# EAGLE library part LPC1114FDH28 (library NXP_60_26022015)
32-bit ARM Cortex-M0 microcontroller; up to 64 kB flash and 8 kB SRAM The LPC1110/11/12/13/14/15 are a ARM Cortex-M0 based, low-cost 32-bit MCU family, designed for 8/16-bit microcontroller applications, offering performance, low power, simple instruction set and memory addressing together with reduced code size compared to existing 8/16-bit architectures. The LPC1110/11/12/13/14/15 operate at CPU frequencies of up to 50 MHz. The peripheral complement of the LPC1110/11/12/13/14/15 includes up to 64 kB of flash memory, up to 8 kB of data memory, one Fast-mode Plus I 2 C-bus interface, one RS-485/EIA-485 UART, up to two SPI interfaces with SSP features, four general purpose counter/timers, a 10-bit ADC, and up to 42 general purpose I/O pins. Remark: The LPC111x series consists of the LPC1100 series (parts LPC111x/101/201/301), LPC1100L series (parts LPC111x/002/102/202/302), and the LPC1100XL series (parts LPC111x/103/203/303/323/333). The LPC1100L and LPC1100XL series include the power profiles, a windowed watchdog timer, and a configurable open-drain mode. AAL Eindhoven MK
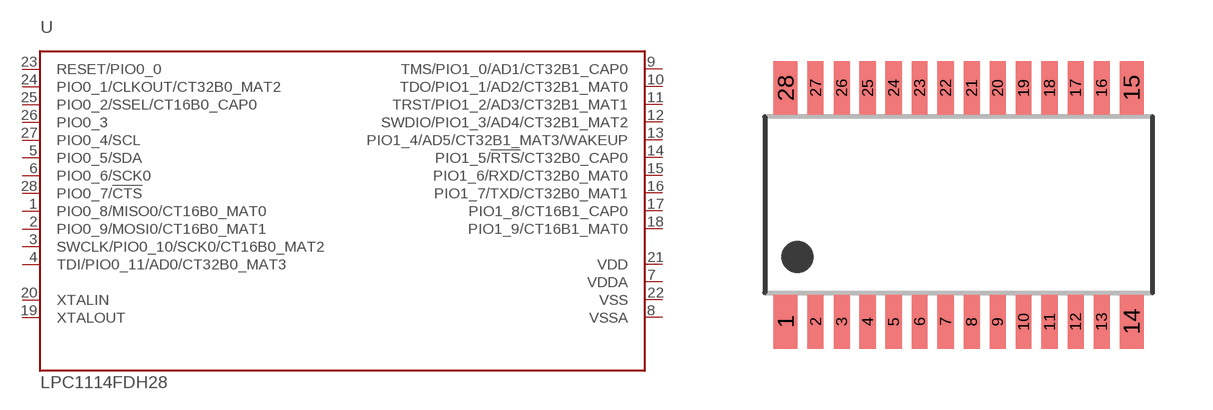
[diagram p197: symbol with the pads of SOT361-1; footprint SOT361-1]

Designator prefix U

## LPC1114FDH28/102 (ADC: 6; FLASH: 32kB; GPIO: 22; PWR_PROFILES: yes; SERIES: LPC1100L; SPI: 1; SRAM: 4kB)  [SOT361-1]
1  PIO0_8/MISO0/CT16B0_MAT0
2  PIO0_9/MOSI0/CT16B0_MAT1
3  SWCLK/PIO0_10/SCK0/CT16B0_MAT2
4  TDI/PIO0_11/AD0/CT32B0_MAT3
5  PIO0_5/SDA
6  PIO0_6/SCK0
7  VDDA  pwr
8  VSSA  pwr
9  TMS/PIO1_0/AD1/CT32B1_CAP0
10  TDO/PIO1_1/AD2/CT32B1_MAT0
11  TRST/PIO1_2/AD3/CT32B1_MAT1
12  SWDIO/PIO1_3/AD4/CT32B1_MAT2
13  PIO1_4/AD5/CT32B1_MAT3/WAKEUP
14  PIO1_5/!RTS!/CT32B0_CAP0
15  PIO1_6/RXD/CT32B0_MAT0
16  PIO1_7/TXD/CT32B0_MAT1
17  PIO1_8/CT16B1_CAP0
18  PIO1_9/CT16B1_MAT0
19  XTALOUT  out
20  XTALIN  in
21  VDD  pwr
22  VSS  pwr
23  RESET/PIO0_0
24  PIO0_1/CLKOUT/CT32B0_MAT2
25  PIO0_2/SSEL/CT16B0_CAP0
26  PIO0_3
27  PIO0_4/SCL
28  PIO0_7/!CTS!

## Footprint SOT361-1 (pad centres in mm)
SOT361-1 TSSOP28: plastic thin shrink small outline package; 28 leads; body width 4.4 mm JEDEC: MO-153 IEC: ---
smd 0.6 x 1.35: 1 -4.325,-2.925; 14 4.325,-2.925; 15 4.325,2.925; 28 -4.325,2.925
smd 0.4 x 1.35: 2 -3.575,-2.925; 3 -2.925,-2.925; 4 -2.275,-2.925; 5 -1.625,-2.925; 6 -0.975,-2.925; 7 -0.325,-2.925; 8 0.325,-2.925; 9 0.975,-2.925; 10 1.625,-2.925; 11 2.275,-2.925; 12 2.925,-2.925; 13 3.575,-2.925; 16 3.575,2.925; 17 2.925,2.925; 18 2.275,2.925; 19 1.625,2.925; 20 0.975,2.925; 21 0.325,2.925; 22 -0.325,2.925; 23 -0.975,2.925; 24 -1.625,2.925; 25 -2.275,2.925; 26 -2.925,2.925; 27 -3.575,2.925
